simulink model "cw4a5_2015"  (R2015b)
settings: Solver=FixedStepAuto  SolverMode=SingleTasking  StartTime=0.0  StopTime=100  FixedStep=0.01  RelTol=1e-3
libraries: neural x38, simulink x1

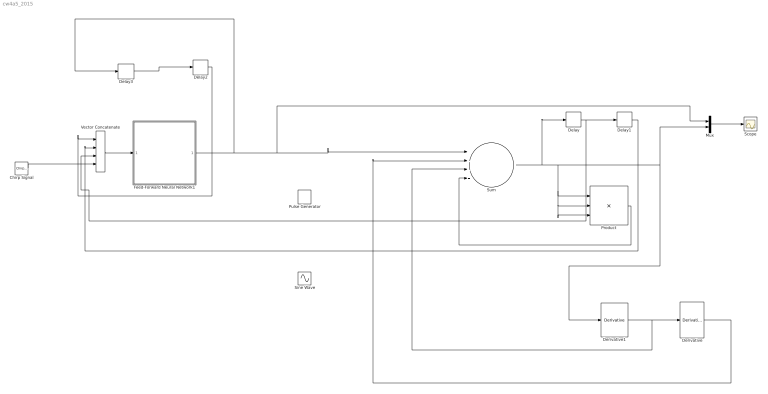
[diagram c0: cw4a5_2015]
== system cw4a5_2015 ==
  Chirp Signal : simulink/Sources/Chirp Signal  f1=0.02  T=100  f2=0.2
  Delay{,1..3} (4 alike) : Delay  DelayLength=1  InitialCondition=0
  Derivative : Derivative
  Derivative1 : Derivative
  Feed-Forward Neural Network1 : Subsystem
  Mux : Mux  Inputs=2
  Product : Product  Inputs=3
  Pulse Generator : DiscretePulseGenerator  PulseType=Time based  Period=10  PulseWidth=50
  Scope : Scope
  Sine Wave : Sin  Frequency=0.11  SampleTime=0
  Sum : Sum  Inputs=+---
  Vector Concatenate : Concatenate  NumInputs=4
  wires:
  Vector Concatenate/1 -> Feed-Forward Neural Network1/1(Input)
  Mux/1 -> Scope/1
  Product/1 -> Sum/4
  Sum/1 -> Delay/1, Product/2, Product/3, Product/1, Derivative1/1, Mux/2
  Derivative1/1 -> Sum/3, Derivative/1
  Derivative/1 -> Sum/2
  Chirp Signal/1 -> Vector Concatenate/4
  Delay/1 -> Delay1/1, Vector Concatenate/3
  Feed-Forward Neural Network1/1(Output) -> Delay3/1, Mux/1, Sum/1
  Delay3/1 -> Delay2/1
  Delay1/1 -> Vector Concatenate/2
  Delay2/1 -> Vector Concatenate/1

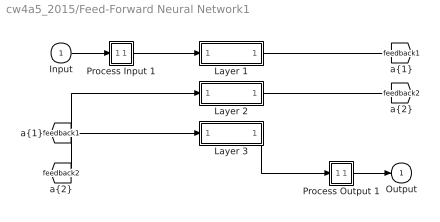
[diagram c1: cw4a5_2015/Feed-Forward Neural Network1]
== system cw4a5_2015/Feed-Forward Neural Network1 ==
  Input : Inport  PortDimensions=4  SampleTime=0.01
  Layer 1 : Subsystem
  Layer 2 : Subsystem
  Layer 3 : Subsystem
  Process Input 1 : Subsystem
  Process Output 1 : Subsystem
  Output : Outport  InitialOutput=0
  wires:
  Input/1 -> Process Input 1/1(x)
  Process Output 1/1(y) -> Output/1
  Process Input 1/1(p) -> Layer 1/1("p{1}")
  Layer 1/1("a{1}") -> [feedback1]
  [feedback1] -> Layer 2/1("a{1} ")
  Layer 2/1("a{2}") -> [feedback2]
  [feedback2] -> Layer 3/1("a{2} ")
  Layer 3/1("a{3}") -> Process Output 1/1(a)

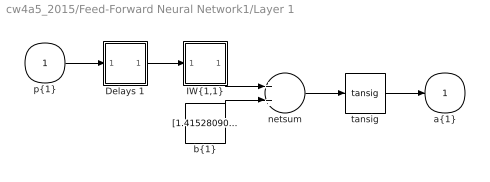
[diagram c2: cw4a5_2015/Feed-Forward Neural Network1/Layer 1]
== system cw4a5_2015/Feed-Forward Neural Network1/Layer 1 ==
  "p{1}" : Inport  PortDimensions=4  SampleTime=0.01
  Delays 1 : Subsystem
  "IW{1,1}" : Subsystem
  "b{1}" : Constant  Value=[1.4152809069992034;-1.9524064234078189;-2.5428224898832679;-2.1299483748619585;-0.47314262609180829;-1.1886995937082012;1.4492996611482065;0.59441971619295619;0.049979498173296152;0.63119747421379313;0.087939147115730795;-2.2514837820737692;-1.8329918316876324;-1.8629583954055342;-2.6727067313361972;-3.2397936113706876]
  netsum : Sum  Inputs=2
  tansig : neural/Transfer Functions/tansig
  "a{1}" : Outport  InitialOutput=[0;0;0;0;0;0;0;0;0;0;0;0;0;0;0;0]
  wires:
  "p{1}"/1 -> Delays 1/1("p{1}")
  Delays 1/1("pd{1,1}") -> "IW{1,1}"/1("pd{1,1}")
  "IW{1,1}"/1("iz{1,1}") -> netsum/1
  "b{1}"/1 -> netsum/2
  netsum/1 -> tansig/1
  tansig/1 -> "a{1}"/1

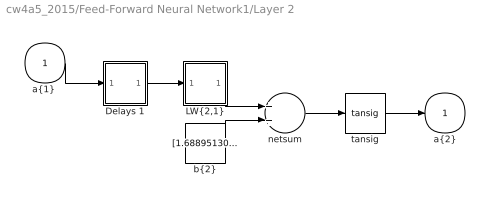
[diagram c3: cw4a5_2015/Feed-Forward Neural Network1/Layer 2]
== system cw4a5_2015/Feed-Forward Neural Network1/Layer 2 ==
  "a{1} " : Inport  PortDimensions=16  SampleTime=0.01
  Delays 1 : Subsystem
  "LW{2,1}" : Subsystem
  "b{2}" : Constant  Value=[1.688951305324133;-1.5407193547140121;1.1180157277577119;-1.0594965123822075;0.50615694433423242;0.34218565659237027;-0.078936347477291377;0.16090870555236744;0.37032700728532614;-0.35923342004397868;-0.55333667818117771;-0.74093603342535308;0.82819566261812194;-1.3650070407799197;1.5494577780860426;1.7109778923912953]
  netsum : Sum  Inputs=2
  tansig : neural/Transfer Functions/tansig
  "a{2}" : Outport  InitialOutput=[0;0;0;0;0;0;0;0;0;0;0;0;0;0;0;0]
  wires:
  "a{1} "/1 -> Delays 1/1("p{2}")
  Delays 1/1("pd{2,1}") -> "LW{2,1}"/1("ad{2,1}")
  "LW{2,1}"/1("lz{2,1}") -> netsum/1
  "b{2}"/1 -> netsum/2
  netsum/1 -> tansig/1
  tansig/1 -> "a{2}"/1

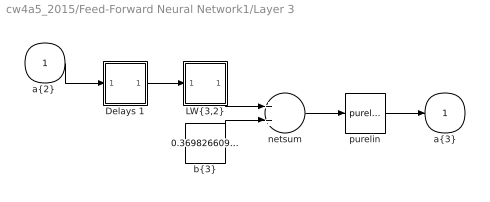
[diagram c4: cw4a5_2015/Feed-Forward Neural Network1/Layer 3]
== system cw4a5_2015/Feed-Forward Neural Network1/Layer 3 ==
  "a{2} " : Inport  PortDimensions=16  SampleTime=0.01
  Delays 1 : Subsystem
  "LW{3,2}" : Subsystem
  "b{3}" : Constant  Value=0.36982660912907933
  netsum : Sum  Inputs=2
  purelin : neural/Transfer Functions/purelin
  "a{3}" : Outport  InitialOutput=0
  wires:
  "a{2} "/1 -> Delays 1/1("p{3}")
  Delays 1/1("pd{3,2}") -> "LW{3,2}"/1("ad{3,2}")
  "LW{3,2}"/1("lz{3,2}") -> netsum/1
  "b{3}"/1 -> netsum/2
  netsum/1 -> purelin/1
  purelin/1 -> "a{3}"/1

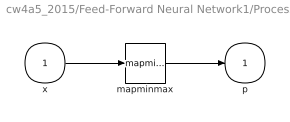
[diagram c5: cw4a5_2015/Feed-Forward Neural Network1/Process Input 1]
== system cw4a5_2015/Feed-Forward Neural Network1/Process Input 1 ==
  x : Inport  PortDimensions=4  SampleTime=0.01
  mapminmax : neural/Processing Functions/mapminmax  xmin=[-0.99999994897995692;-0.8715984089430312;-0.8715984089430312;-0.8715984089430312]  xmax=[1;0.87243553228952253;0.87243553228952253;0.87243553228952253]  ymin=-1  ymax=1
  p : Outport  PortDimensions=4  SampleTime=0.01
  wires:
  x/1 -> mapminmax/1
  mapminmax/1 -> p/1

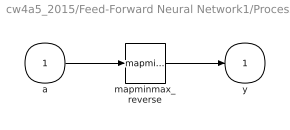
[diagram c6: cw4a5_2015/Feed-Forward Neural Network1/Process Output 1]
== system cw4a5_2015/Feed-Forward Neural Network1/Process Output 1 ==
  a : Inport  PortDimensions=1  SampleTime=0.01
  mapminmax_reverse : neural/Processing Functions/mapminmax_reverse  xmin=-0.99999994897995692  xmax=1  ymin=-1  ymax=1
  y : Outport  PortDimensions=1  SampleTime=0.01
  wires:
  a/1 -> mapminmax_reverse/1
  mapminmax_reverse/1 -> y/1

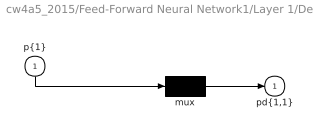
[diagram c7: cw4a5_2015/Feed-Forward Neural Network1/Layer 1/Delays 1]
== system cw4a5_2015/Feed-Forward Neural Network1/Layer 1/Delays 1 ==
  "p{1}" : Inport  PortDimensions=4  SampleTime=0.01
  mux : Mux  Inputs=1
  "pd{1,1}" : Outport
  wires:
  "p{1}"/1 -> mux/1
  mux/1 -> "pd{1,1}"/1

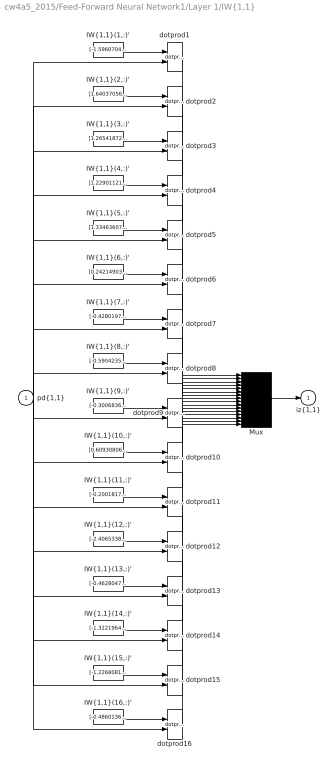
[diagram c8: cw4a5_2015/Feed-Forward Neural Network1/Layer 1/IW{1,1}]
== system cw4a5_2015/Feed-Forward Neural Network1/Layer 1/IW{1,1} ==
  "pd{1,1}" : Inport  PortDimensions=4  SampleTime=0.01
  "IW{1,1}(1,:)'" : Constant  Value=[-1.5960704613459544;1.4687532103356533;-0.77344391577477389;1.144204952184015]
  "IW{1,1}(10,:)'" : Constant  Value=[0.609308069330741;1.8437098054485526;1.4716126103591822;-0.87145490986372087]
  "IW{1,1}(11,:)'" : Constant  Value=[-0.20018179296029573;-3.991167139448045;0.060818934404480759;3.4715825212576239]
  "IW{1,1}(12,:)'" : Constant  Value=[-2.4065338050635234;1.083276561370133;2.9647780135264594;1.2312854423506749]
  "IW{1,1}(13,:)'" : Constant  Value=[-0.46280475466442572;-0.24869793706538412;-0.64326687846050734;-2.3021258939269043]
  "IW{1,1}(14,:)'" : Constant  Value=[-1.3221964113101545;2.5000772033777423;-0.34636845314331061;-1.0476855440342734]
  "IW{1,1}(15,:)'" : Constant  Value=[-1.2268081488282436;-0.60508936441403027;-1.8315057370272536;1.3944386302669998]
  "IW{1,1}(16,:)'" : Constant  Value=[-0.48601369820675827;-1.9361678790251415;-1.1284692009618027;-0.45583588617638776]
  "IW{1,1}(2,:)'" : Constant  Value=[1.640370568885146;1.2928514670750937;0.4677877221829666;0.37388339470195525]
  "IW{1,1}(3,:)'" : Constant  Value=[1.2654187234764194;0.76077003385776099;-1.6730375742583723;1.3974089654228536]
  "IW{1,1}(4,:)'" : Constant  Value=[1.2290112141762262;1.3287484123203408;-1.5579712029031474;1.4044485301153191]
  "IW{1,1}(5,:)'" : Constant  Value=[1.3346360713408252;1.4615193004083702;-1.2284436104033805;-2.4091423668227758]
  "IW{1,1}(6,:)'" : Constant  Value=[0.24214903430169055;-1.4766940079813911;1.5096611864588765;-1.9425053052009591]
  "IW{1,1}(7,:)'" : Constant  Value=[-0.42801978197827306;-2.0139459914204192;-1.7826752957064644;1.4708922911867395]
  "IW{1,1}(8,:)'" : Constant  Value=[-0.59042352420562028;-1.07305482263509;-1.4079824855198357;0.14080262886023334]
  "IW{1,1}(9,:)'" : Constant  Value=[-0.30068367490993947;1.4890658067029769;1.9064042289111662;-3.4521609371185367]
  Mux : Mux  Inputs=16
  dotprod{1..16} (16 alike) : neural/Weight Functions/dotprod
  "iz{1,1}" : Outport
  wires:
  "IW{1,1}(1,:)'"/1 -> dotprod1/1
  "pd{1,1}"/1 -> dotprod1/2, dotprod2/2, dotprod3/2, dotprod4/2, dotprod5/2, dotprod6/2, dotprod7/2, dotprod8/2, dotprod9/2, dotprod10/2, dotprod11/2, dotprod12/2, dotprod13/2, dotprod14/2, dotprod15/2, dotprod16/2
  dotprod1/1 -> Mux/1
  "IW{1,1}(2,:)'"/1 -> dotprod2/1
  dotprod2/1 -> Mux/2
  "IW{1,1}(3,:)'"/1 -> dotprod3/1
  dotprod3/1 -> Mux/3
  "IW{1,1}(4,:)'"/1 -> dotprod4/1
  dotprod4/1 -> Mux/4
  "IW{1,1}(5,:)'"/1 -> dotprod5/1
  dotprod5/1 -> Mux/5
  "IW{1,1}(6,:)'"/1 -> dotprod6/1
  dotprod6/1 -> Mux/6
  "IW{1,1}(7,:)'"/1 -> dotprod7/1
  dotprod7/1 -> Mux/7
  "IW{1,1}(8,:)'"/1 -> dotprod8/1
  dotprod8/1 -> Mux/8
  "IW{1,1}(9,:)'"/1 -> dotprod9/1
  dotprod9/1 -> Mux/9
  "IW{1,1}(10,:)'"/1 -> dotprod10/1
  dotprod10/1 -> Mux/10
  "IW{1,1}(11,:)'"/1 -> dotprod11/1
  dotprod11/1 -> Mux/11
  "IW{1,1}(12,:)'"/1 -> dotprod12/1
  dotprod12/1 -> Mux/12
  "IW{1,1}(13,:)'"/1 -> dotprod13/1
  dotprod13/1 -> Mux/13
  "IW{1,1}(14,:)'"/1 -> dotprod14/1
  dotprod14/1 -> Mux/14
  "IW{1,1}(15,:)'"/1 -> dotprod15/1
  dotprod15/1 -> Mux/15
  "IW{1,1}(16,:)'"/1 -> dotprod16/1
  dotprod16/1 -> Mux/16
  Mux/1 -> "iz{1,1}"/1

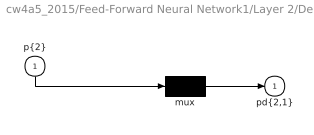
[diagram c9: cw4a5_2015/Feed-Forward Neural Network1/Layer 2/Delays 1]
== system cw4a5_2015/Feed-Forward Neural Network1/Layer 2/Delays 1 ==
  "p{2}" : Inport  PortDimensions=16  SampleTime=0.01
  mux : Mux  Inputs=1
  "pd{2,1}" : Outport
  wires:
  "p{2}"/1 -> mux/1
  mux/1 -> "pd{2,1}"/1

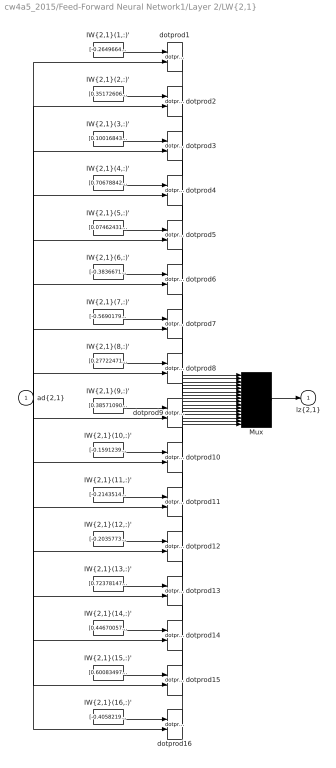
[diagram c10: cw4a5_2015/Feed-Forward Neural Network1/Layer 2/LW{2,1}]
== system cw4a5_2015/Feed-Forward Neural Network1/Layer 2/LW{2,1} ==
  "ad{2,1}" : Inport  PortDimensions=16  SampleTime=0.01
  "IW{2,1}(1,:)'" : Constant  Value=[-0.26496640782118386;0.61102658560270207;-0.15871792485394151;-0.63273552338370487;0.4360346547575108;0.82587647633477113;0.70478959716343847;0.01534788839966549;-0.96063788526770788;0.10725265383197247;-0.17977416945967029;0.24077348285801206;0.20106959322584891;0.32231787209218715;0.2837700347509664;0.22408635263416898]
  "IW{2,1}(10,:)'" : Constant  Value=[-0.15912396380284743;-0.25038382242744267;0.085856587498447851;0.599986386922846;-0.60666517385127461;0.47093389749917025;0.23457318663666338;0.18990339591840691;-0.69614307481121751;-0.35152354800478963;1.1565644346014055;0.27947157240132037;-0.034511753680713714;0.63932256810393617;0.41361358876558352;-0.46263725565232677]
  "IW{2,1}(11,:)'" : Constant  Value=[-0.21435144647231177;-0.13199210470017081;0.48564180337837498;-0.45124984809276597;0.64471867237288227;0.33492033766503188;0.073041979775123209;0.40933349165726995;-0.66709626976882752;-0.47753901781272473;-0.3908627684931425;-0.66358149246707476;0.0053492095086546277;-0.19397200163779327;0.97732366340317478;0.61544215913170464]
  "IW{2,1}(12,:)'" : Constant  Value=[-0.2035773025396834;0.65644356715054286;0.33184277025539227;-0.30397004539988526;-0.038435087933637334;0.57447107518948437;-0.39098474894704377;-0.67101297310506258;-0.71767280452483773;0.10024505967536182;1.0891054333262009;-0.38443717379230746;0.7084150997153762;0.63373410628790416;-0.20821178167185464;-0.16230310233162909]
  "IW{2,1}(13,:)'" : Constant  Value=[0.72378147661212033;0.027997259658700965;-0.95120021592736492;-0.3286199331325152;0.43134052134277578;-0.47447791418008822;0.18230664692222501;0.58075268122670964;1.4624876523152546;-0.64888046774017138;0.83259390473120598;-0.080333529416052249;-0.20126012998913881;0.29470027754654898;0.52901064426700839;-0.4310033918176851]
  "IW{2,1}(14,:)'" : Constant  Value=[0.44670057377386346;-0.17595846198329043;-0.41413464690603996;0.088570699018922047;-0.27098599538461793;0.48732878781447825;-0.17072090693118319;0.070441925816825471;0.51122140952934214;0.617580173660359;0.67652492419818477;-0.048438786344837559;0.31968397497334072;-0.27331734028553295;-0.7275051968926296;-0.28633180038134526]
  "IW{2,1}(15,:)'" : Constant  Value=[0.60083497342247449;-0.62575861463458982;-0.09052782297984463;0.67660160893549248;-0.69399859678265274;-0.54627777230101315;0.084833746096537113;0.68121287850773493;0.68622934167756511;-0.47916614283277276;0.11100445763973132;0.48867589597675809;0.31789262979710498;-0.14818457513424882;0.072364962821976214;-0.26859835657808689]
  "IW{2,1}(16,:)'" : Constant  Value=[-0.40582190298042753;0.48336419434623279;0.38547173278379093;0.21367770937814096;0.4610182617147246;0.32044419021604814;-0.47071406599992199;-0.21673750862973423;0.61152931666212695;0.44783946689956355;1.1034679057644996;0.23952606162808554;-0.69388608442794819;-0.81390904706147627;-0.22370357303876295;0.73885001026082575]
  "IW{2,1}(2,:)'" : Constant  Value=[0.35172606827624403;-0.20312028687283443;-0.92510915497987134;-0.79782293587855502;1.0036975887601318;0.1111179225971814;-1.5820463278448127;-0.10420986770616138;-1.0086204765009592;-0.70648223393458986;0.31703949882015819;-0.5066982139568853;-0.07824007040614403;-0.38471145943247287;0.016588822635293571;1.1065817747421276]
  "IW{2,1}(3,:)'" : Constant  Value=[0.10016843590592039;-0.036028925667805231;-0.070232716705176335;0.91754509028510201;1.0419119480310577;0.65625679856180141;-1.0658257955690558;-0.041393050042536968;0.42947175932428705;-0.17351226039785439;1.276323488920494;0.16354045214480167;-0.28282876502524068;-0.56315123912675658;0.35862424018353828;0.7021319558249185]
  "IW{2,1}(4,:)'" : Constant  Value=[0.70678842020973198;0.40439292056986964;0.65928929107272893;-0.59068370909280621;-0.84525071424516995;0.75059112563428543;-0.16890444618988684;-0.05152889182014174;-0.069289446847533187;0.11635122813016546;0.11001835859323696;-0.5203459996204054;0.77886806330524883;0.72243724779198182;0.2176792199764945;0.23874403365511726]
  "IW{2,1}(5,:)'" : Constant  Value=[0.074624314965116831;0.11192765856089958;0.18278417741522696;0.9205790937917514;0.37366352156404176;-0.65103305320509153;0.056845682274251332;-0.20505848106199812;1.1113384010213736;-0.29839316018555501;0.79983569794074116;0.022467322083626558;-0.35682718488773013;0.20410808759501825;0.1697979900407145;0.17426595483506258]
  "IW{2,1}(6,:)'" : Constant  Value=[-0.38366719964313689;-0.45185000569645012;0.34310018336928533;0.12756035941569632;-0.24751399622140421;0.22969355968098984;0.52275331844596917;0.13393544776753616;1.3016211036028134;-0.1047880834361085;-0.17216254269456369;-0.1016964242188543;0.16077208928816883;0.12191710741138834;0.57256922261263299;-0.10611150743568414]
  "IW{2,1}(7,:)'" : Constant  Value=[-0.56901794852060139;0.12291007132669975;0.72576679118225429;0.095393354016622578;-0.90995363459778433;0.34254733232480039;-0.043295609053622806;-0.035139176604380221;-0.18490419354010879;0.85283952817459652;0.78046938257229714;0.14850064701685922;0.09030611585672095;0.70577668394144655;-0.10506222131685584;-0.1159229170323389]
  "IW{2,1}(8,:)'" : Constant  Value=[0.27722471405095378;-0.62455240298399828;-0.56403793043284245;0.73614310046645637;-0.59258777400527685;0.12367758036522331;-0.16061781105296752;0.49733435959504224;-0.57867040951483961;-0.89568242629736128;0.38909753195080266;-0.21254415731326717;-0.086289135244234275;0.0095706716946589443;-0.10402128906002789;-0.71409449688117421]
  "IW{2,1}(9,:)'" : Constant  Value=[0.3857109069948606;-0.57242561411983295;0.16417347147962588;0.24920542908154861;-0.25055804124829834;0.39824975115919115;-0.27296714276488571;-0.20683651385023152;-0.0045754546946230358;0.49819773316020449;-1.1877125899136951;-0.23584380081440862;-0.37070901748129764;-0.62474602451160788;-0.015289443260539458;0.21375968854837279]
  Mux : Mux  Inputs=16
  dotprod{1..16} (16 alike) : neural/Weight Functions/dotprod
  "lz{2,1}" : Outport
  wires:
  "IW{2,1}(1,:)'"/1 -> dotprod1/1
  "ad{2,1}"/1 -> dotprod1/2, dotprod2/2, dotprod3/2, dotprod4/2, dotprod5/2, dotprod6/2, dotprod7/2, dotprod8/2, dotprod9/2, dotprod10/2, dotprod11/2, dotprod12/2, dotprod13/2, dotprod14/2, dotprod15/2, dotprod16/2
  dotprod1/1 -> Mux/1
  "IW{2,1}(2,:)'"/1 -> dotprod2/1
  dotprod2/1 -> Mux/2
  "IW{2,1}(3,:)'"/1 -> dotprod3/1
  dotprod3/1 -> Mux/3
  "IW{2,1}(4,:)'"/1 -> dotprod4/1
  dotprod4/1 -> Mux/4
  "IW{2,1}(5,:)'"/1 -> dotprod5/1
  dotprod5/1 -> Mux/5
  "IW{2,1}(6,:)'"/1 -> dotprod6/1
  dotprod6/1 -> Mux/6
  "IW{2,1}(7,:)'"/1 -> dotprod7/1
  dotprod7/1 -> Mux/7
  "IW{2,1}(8,:)'"/1 -> dotprod8/1
  dotprod8/1 -> Mux/8
  "IW{2,1}(9,:)'"/1 -> dotprod9/1
  dotprod9/1 -> Mux/9
  "IW{2,1}(10,:)'"/1 -> dotprod10/1
  dotprod10/1 -> Mux/10
  "IW{2,1}(11,:)'"/1 -> dotprod11/1
  dotprod11/1 -> Mux/11
  "IW{2,1}(12,:)'"/1 -> dotprod12/1
  dotprod12/1 -> Mux/12
  "IW{2,1}(13,:)'"/1 -> dotprod13/1
  dotprod13/1 -> Mux/13
  "IW{2,1}(14,:)'"/1 -> dotprod14/1
  dotprod14/1 -> Mux/14
  "IW{2,1}(15,:)'"/1 -> dotprod15/1
  dotprod15/1 -> Mux/15
  "IW{2,1}(16,:)'"/1 -> dotprod16/1
  dotprod16/1 -> Mux/16
  Mux/1 -> "lz{2,1}"/1

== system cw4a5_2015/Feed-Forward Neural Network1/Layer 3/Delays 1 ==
  "p{3}" : Inport  PortDimensions=16  SampleTime=0.01
  mux : Mux  Inputs=1
  "pd{3,2}" : Outport
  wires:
  "p{3}"/1 -> mux/1
  mux/1 -> "pd{3,2}"/1

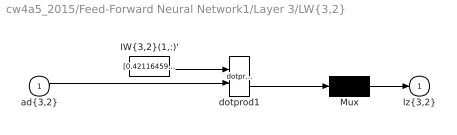
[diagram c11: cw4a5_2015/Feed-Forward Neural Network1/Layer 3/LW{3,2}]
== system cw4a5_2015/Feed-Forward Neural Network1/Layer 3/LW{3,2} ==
  "ad{3,2}" : Inport  PortDimensions=16  SampleTime=0.01
  "IW{3,2}(1,:)'" : Constant  Value=[0.42116459332705014;1.3527672604817524;-1.6043738797708484;-0.82296681213774414;-1.3685100536357524;-0.89821977634500016;-0.50208635421237335;0.33083366498967459;0.94401140256980887;0.6453745259314676;0.99806984798461085;-1.0555905363771485;-2.305561502930821;-1.0849907842820299;-0.36559931979084531;-0.74788442712759784]
  Mux : Mux  Inputs=1
  dotprod1 : neural/Weight Functions/dotprod
  "lz{3,2}" : Outport
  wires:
  "IW{3,2}(1,:)'"/1 -> dotprod1/1
  "ad{3,2}"/1 -> dotprod1/2
  dotprod1/1 -> Mux/1
  Mux/1 -> "lz{3,2}"/1
